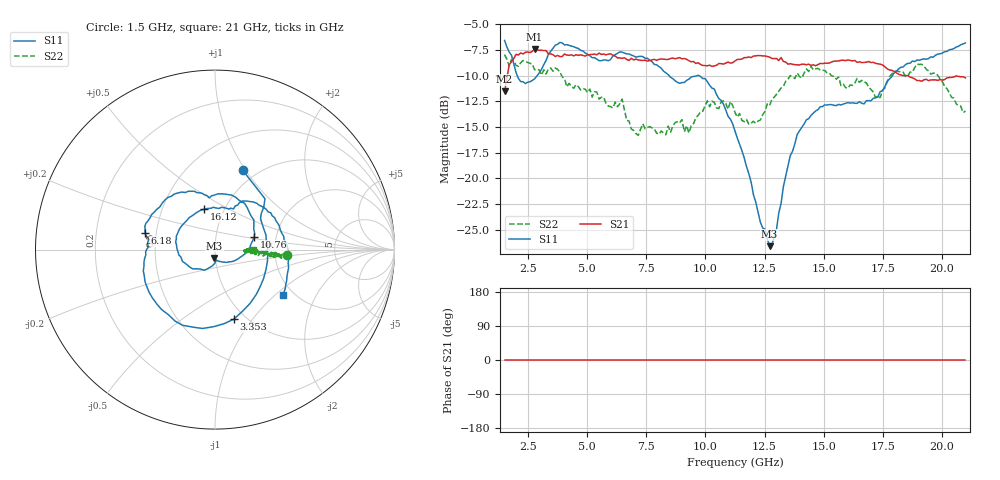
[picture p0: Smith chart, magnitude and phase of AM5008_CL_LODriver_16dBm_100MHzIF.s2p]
!Keysight Technologies,N5245B,MY58422270,A.16.20.02
!Mixer S2P File: Scalar Mixer Measurement
!Calibration State: On
!Parameters: Stimulus Freq, S11, SC21, SC12, S22
# Hz  S  DB  R  50.0
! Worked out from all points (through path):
!   201 points, 1.5 GHz to 21 GHz, reference 50 ohm
!   highest |S21| = -7.42 dB at 2.768 GHz (marker M1); lowest = -11.5 dB at 1.5 GHz (marker M2)
!   lowest |S11| = -26.6 dB at 12.71 GHz (marker M3), VSWR 1.10, Z = 49.4 - j4.61 ohm
!   |S11| at or under -10 dB: 2.036 GHz to 2.879 GHz (842.4 MHz wide, 34.3 % of centre); 8.46 GHz to 9.648 GHz (1.187 GHz wide, 13.1 % of centre); 9.72 GHz to 17.91 GHz (8.19 GHz wide, 59.3 % of centre)
!   |S22| runs from -15.8 to -8.0 dB; largest |S21 - S12| = 0.43
!   S11 on the Smith chart (normalised r, x): 1.5 GHz: 0.86, +0.97; 3.353 GHz: 0.88, -0.82; 6.18 GHz: 0.43, +0.10; 10.76 GHz: 1.54, +0.23; 16.12 GHz: 0.80, +0.38; 21 GHz: 1.76, -1.13
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1.5e9  -6.58 70.8  -11.54 0.0  -200.00 90.0  -7.96 -4.5
1.9875e9  -9.72 37.9  -7.93 0.0  -200.00 90.0  -9.01 -5.9
2.7675e9  -10.32 -21.3  -7.42 0.0  -200.00 90.0  -9.42 -6.2
3.3525e9  -7.93 -74.7  -7.88 0.0  -200.00 90.0  -9.35 -4.2
3.645e9  -7.03 -99.0  -8.15 0.0  -200.00 90.0  -9.26 -5.6
4.1325e9  -6.99 -131.7  -8.00 0.0  -200.00 90.0  -11.09 -2.7
4.815e9  -7.60 -163.5  -8.04 0.0  -200.00 90.0  -11.26 -6.5
6.18e9  -7.95 166.7  -8.09 0.0  -200.00 90.0  -12.59 -1.7
7.155e9  -8.14 138.6  -8.47 0.0  -200.00 90.0  -15.82 -3.5
8.0325e9  -9.12 111.7  -8.41 0.0  -200.00 90.0  -15.71 -3.0
9.69e9  -9.97 73.0  -8.74 0.0  -200.00 90.0  -13.86 -3.5
1.07625e10  -12.78 17.7  -8.87 0.0  -200.00 90.0  -12.48 -3.0
1.125e10  -15.41 -7.7  -8.57 0.0  -200.00 90.0  -13.59 -3.6
1.21275e10  -22.31 -62.4  -8.07 0.0  -200.00 90.0  -14.64 -0.5
1.27125e10  -26.61 -95.2  -8.19 0.0  -200.00 90.0  -12.90 -6.9
1.38825e10  -15.73 -138.8  -8.95 0.0  -200.00 90.0  -9.76 -3.5
1.4565e10  -13.66 -177.5  -8.94 0.0  -200.00 90.0  -9.43 -6.2
1.6125e10  -12.67 105.3  -8.52 0.0  -200.00 90.0  -10.90 -4.0
1.73925e10  -11.57 65.2  -8.89 0.0  -200.00 90.0  -12.15 -5.0
1.77825e10  -10.34 61.1  -9.44 0.0  -200.00 90.0  -10.12 -5.1
1.91475e10  -8.42 22.5  -10.55 0.0  -200.00 90.0  -8.90 -3.9
2.1e10  -6.82 -33.8  -10.21 0.0  -200.00 90.0  -13.46 -1.2
